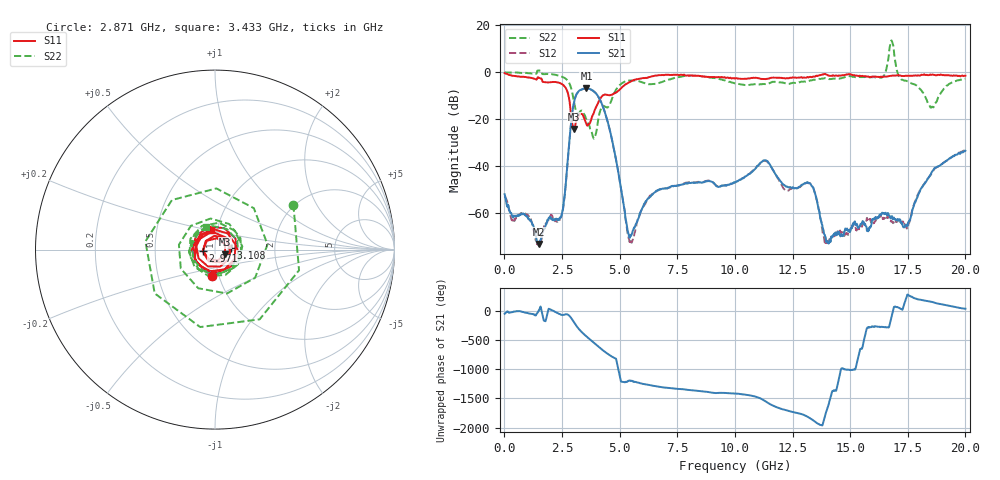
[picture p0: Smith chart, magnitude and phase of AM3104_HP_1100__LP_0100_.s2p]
!Created with skrf (http://scikit-rf.org).
# Hz S RI R 50.0
!freq ReS11 ImS11 ReS21 ImS21 ReS12 ImS12 ReS22 ImS22
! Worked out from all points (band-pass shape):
!   1601 points, 10 MHz to 20 GHz, reference 50 ohm
!   highest |S21| = -6.87 dB at 3.558 GHz (marker M1); lowest = -73.1 dB at 1.497 GHz (marker M2)
!   |S21| within 3 dB of the highest: 3.106 GHz to 4.043 GHz (936.6 MHz wide, 26.2 % of centre)
!   lowest |S11| = -24.2 dB at 3.021 GHz (marker M3), VSWR 1.13, Z = 55.9 - j2.88 ohm
!   |S11| at or under -10 dB: 2.784 GHz to 4.25 GHz (1.466 GHz wide, 41.7 % of centre)
!   |S22| runs from -28.3 to 13.6 dB; largest |S21 - S12| = 0.019
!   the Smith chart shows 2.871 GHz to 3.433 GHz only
!   S11 on the Smith chart (normalised r, x): 2.871 GHz: 0.92, -0.28; 2.971 GHz: 0.87, -0.02; 3.108 GHz: 1.20, +0.03; 3.433 GHz: 0.94, +0.21
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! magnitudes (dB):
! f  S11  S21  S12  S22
! 10 MHz  -0.4  -51.9  -52.8  0.0
! 1.497 GHz  -2.3  -73.1  -73.9  0.8
! 2.471 GHz  -4.8  -61.2  -61.4  -1.8
! 2.871 GHz  -16.6  -23.7  -23.9  -6.0
! 2.971 GHz  -23.1  -15.6  -15.6  -10.0
! 3.021 GHz  -24.2  -12.9  -12.9  -12.6
! 3.108 GHz  -20.9  -9.8  -9.8  -16.5
! 3.346 GHz  -17.7  -7.3  -7.4  -16.3
! 3.433 GHz  -19.0  -7.0  -7.0  -17.3
! 3.558 GHz  -21.9  -6.9  -7.0  -20.1
! 3.896 GHz  -16.8  -8.2  -8.2  -28.1
! 4.433 GHz  -9.6  -19.3  -19.3  -14.9
! 5.445 GHz  -4.1  -70.5  -71.8  -3.5
! 6.682 GHz  -1.2  -50.1  -50.1  -4.6
! 10.01 GHz  -2.7  -46.9  -47.0  -4.7
! 11.32 GHz  -2.9  -37.6  -37.8  -5.0
! 13.34 GHz  -2.0  -48.5  -48.3  -3.4
! 13.98 GHz  -1.0  -72.2  -72.4  -2.7
! 16.68 GHz  -1.6  -61.0  -61.7  7.1
! 17.41 GHz  -1.5  -64.9  -65.3  -3.6
! 18.54 GHz  -1.0  -42.6  -42.8  -14.8
! 20 GHz  -1.4  -33.4  -33.0  -2.7
